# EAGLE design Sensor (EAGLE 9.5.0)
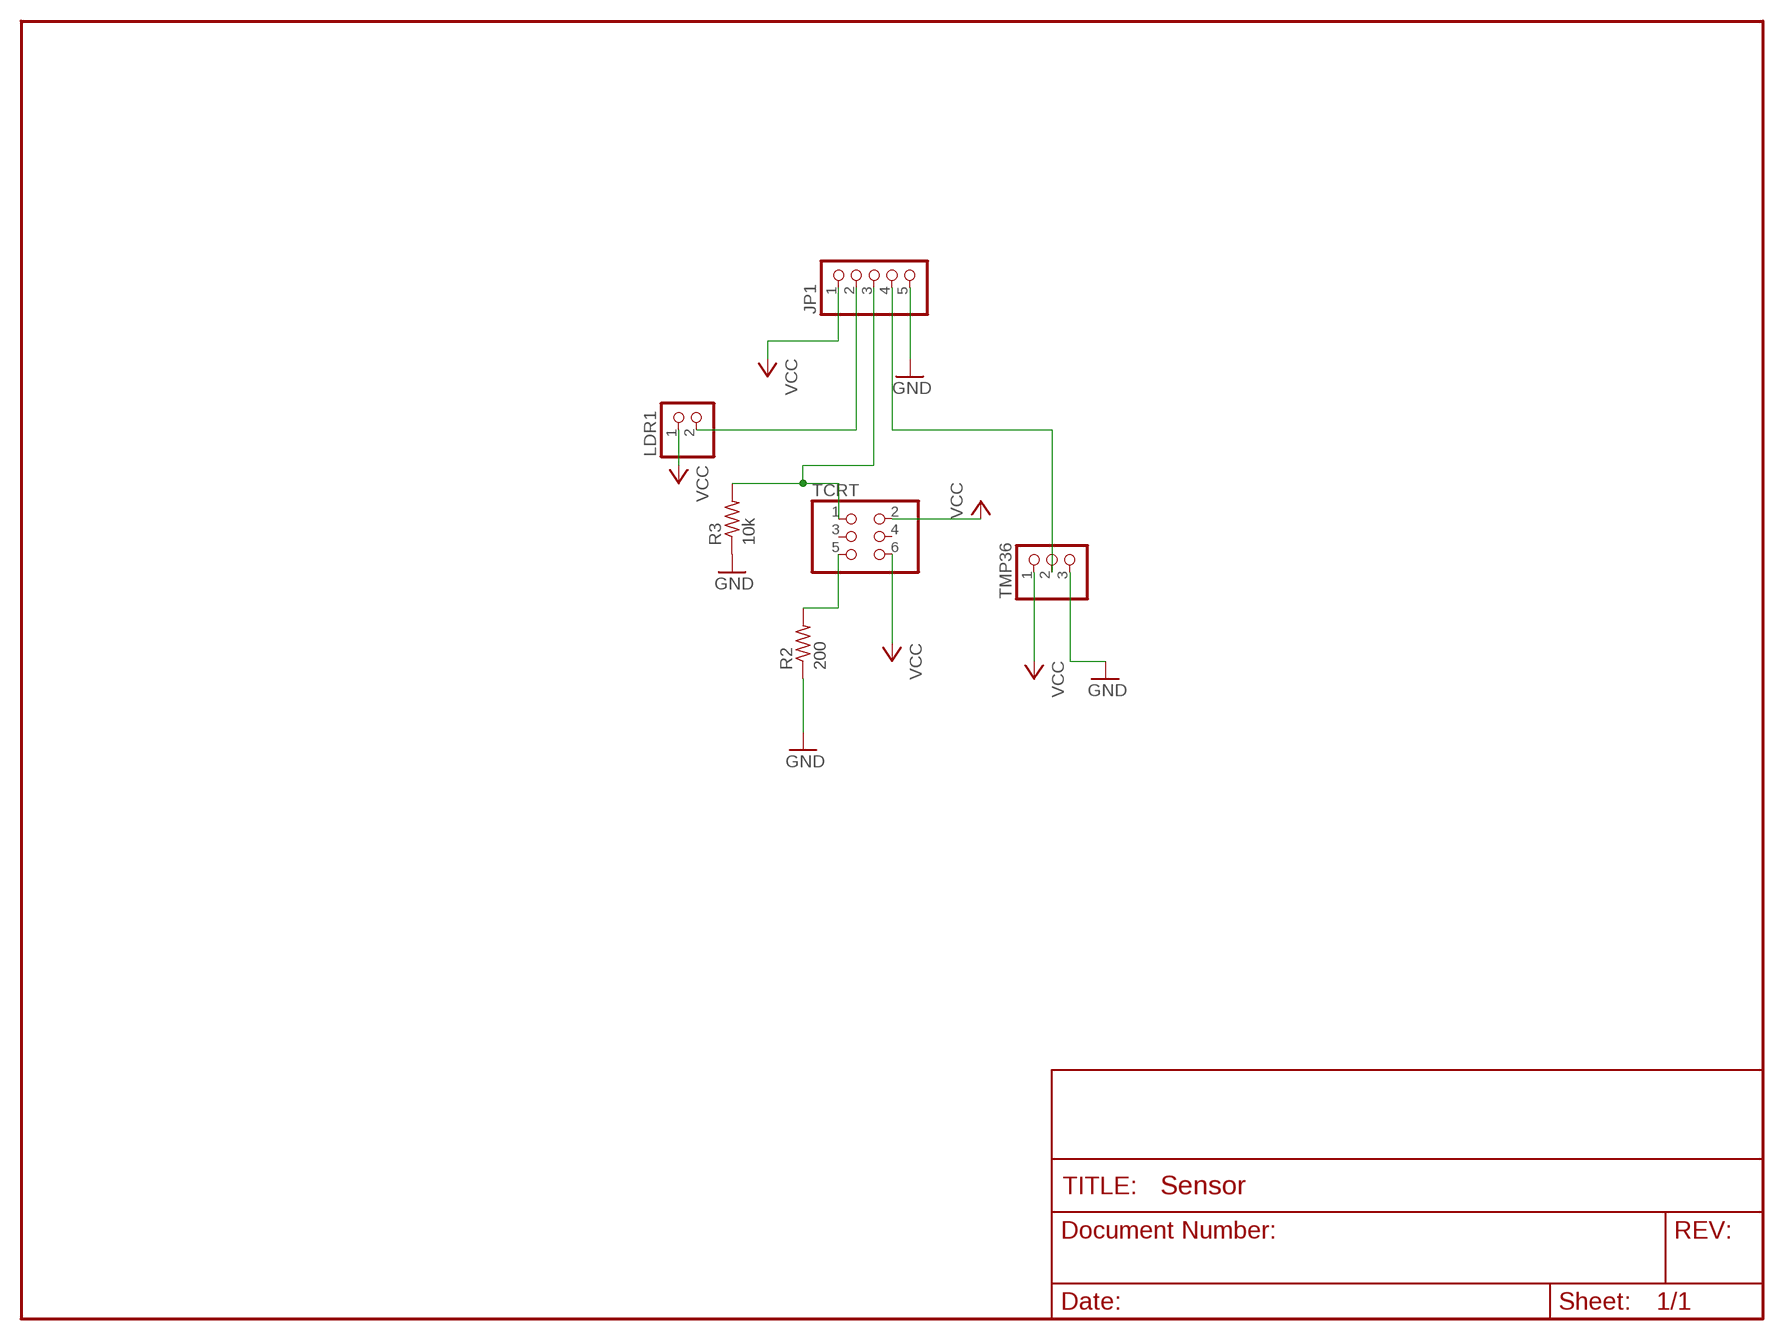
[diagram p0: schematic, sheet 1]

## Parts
JP1  PINHD-1X5  [1X05]
LDR1  PINHD-1X2  [1X02]
R2  200  R-US_0204/5  [0204/5]
R3  10k  R-US_0204/5  [0204/5]
TCRT  PINHD-2X3  [2X03]
TMP36  PINHD-1X3  [1X03]

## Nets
GND [Ground]: JP1.5 R2.1 R3.1 TMP36.3
IR: JP1.3 R3.2 TCRT.1
LDR: JP1.2 LDR1.2
N$1: R2.2 TCRT.5
TEMP: JP1.4 TMP36.2
VCC [Ground]: JP1.1 LDR1.1 TCRT.2 TCRT.6 TMP36.1
Unconnected: TCRT.3 TCRT.4

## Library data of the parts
JP1 = pinhead:PINHD-1X5: PIN HEADER
LDR1 = pinhead:PINHD-1X2: PIN HEADER
R2 R3 = rcl:R-US_: RESISTOR, American symbol; SPICEPREFIX: R
TCRT = pinhead:PINHD-2X3: PIN HEADER
TMP36 = pinhead:PINHD-1X3: PIN HEADER

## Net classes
0 default: width 0.254 mm
1 Power: width 0.508 mm
2 Ground: width 0.508 mm

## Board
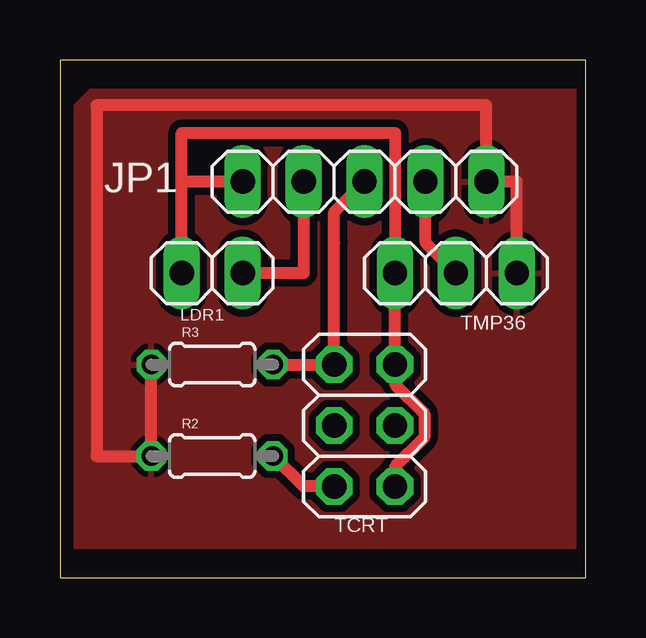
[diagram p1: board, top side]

Size 21.92 x 21.58 mm. Coordinates in mm from the lower left corner, seen from the top.
Outline: 0,0 21.92,0 21.92,21.58 0,21.58 0,0
Copper layers (1*16): Top 0.0356mm / dielectric 1.5011mm / Bottom 0.0356mm
Design rules "ECE_Senior_Design *": minimum track width 8mil, minimum drill 13mil, track to track 8mil, track to pad 8mil, pad to pad 6mil, via to via 8mil, smd to smd 6mil, copper to edge 15mil, drill to drill 8mil, minimum pad ring 7mil, minimum via ring 7mil, stop-mask expansion 3mil, vias tented up to drill 0mil, thermal gap 10mil

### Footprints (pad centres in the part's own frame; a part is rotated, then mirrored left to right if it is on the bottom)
1X05 = drill 1.016 long: 1 -5.08,0; 2 -2.54,0; 3 0,0; 4 2.54,0; 5 5.08,0
1X02 = drill 1.016 long: 1 -1.27,0; 2 1.27,0
0204/5 = drill 0.813 octagon: 1 -2.54,0; 2 2.54,0
2X03 = drill 1.016 octagon: 1 -2.54,-1.27; 2 -2.54,1.27; 3 0,-1.27; 4 0,1.27; 5 2.54,-1.27; 6 2.54,1.27
1X03 = drill 1.016 long: 1 -2.54,0; 2 0,0; 3 2.54,0

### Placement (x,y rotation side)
JP1  12.7,16.51 0 top
LDR1  6.35,12.7 0 top
R2  6.35,5.08 0 top
R3  6.35,8.89 0 top
TCRT  12.7,6.35 270 top
TMP36  16.51,12.7 0 top

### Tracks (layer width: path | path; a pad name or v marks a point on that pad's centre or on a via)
GND
  Top 0.508: TMP36.3 19.05,16.51 JP1.5 17.78,19.68 1.52,19.68 1.52,5.08 R2.1 R3.1
  pour Top (isolate 0.305): 1.27,20.32 21.59,20.32 21.59,1.27 0.63,1.27 0.63,19.68
IR
  Top 0.508: R3.2 TCRT.1 11.43,13.97 11.43,15.24 JP1.3
LDR
  Top 0.508: LDR1.2 10.16,12.7 JP1.2
N$1
  Top 0.508: TCRT.5 10.16,3.81 R2.2
TEMP
  Top 0.508: 16.51,13.97 TMP36.2 15.24,13.97 JP1.4
VCC
  Top 0.508: TCRT.6 13.97,4.63 15.19,5.85 15.19,6.86 13.97,8.07 TCRT.2 TMP36.1 13.97,18.54 5.08,18.54 5.08,16.51 | LDR1.1 5.08,16.51 | JP1.1 5.08,16.51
